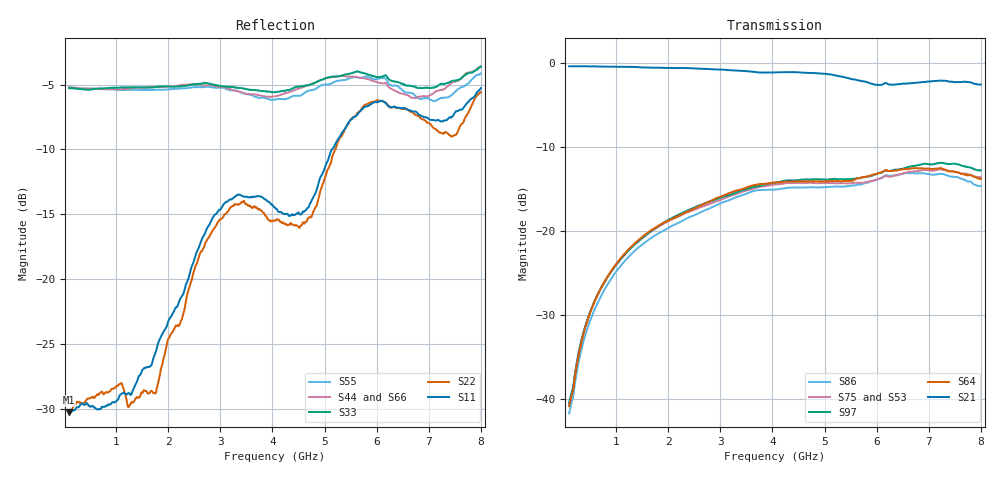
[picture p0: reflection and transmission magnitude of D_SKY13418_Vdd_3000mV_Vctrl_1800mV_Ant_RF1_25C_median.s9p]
# GHz S DB R 50
! THRU S21 mag phase subtraction.
! HALF_THRU
! EN33-165-011-v1_HALF_THRU_1 EN33-165-011-v1_HALF_THRU_2 EN33-165-011-v1_HALF_THRU_3 EN33-165-011-v1_HALF_THRU_4 EN33-165-011-v1_HALF_THRU_5 EN33-165-011-v1_HALF_THRU_6 EN33-165-011-v1_HALF_THRU_7 EN33-165-011-v1_HALF_THRU_8 EN33-165-011-v1_HALF_THRU_9
! THRU Ports: 1 2
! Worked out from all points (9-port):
!   801 points, 100 MHz to 8 GHz, reference 50 ohm
!   strongest paths, dB at 100 MHz, 2.075 GHz, 4.05 GHz, 6.025 GHz, 8 GHz:
!     S21: -0.4, -0.6, -1.1, -2.6, -2.5
!     S64: -40.8, -18.5, -14.2, -13.1, -13.8
!     S97: -40.5, -18.4, -14.2, -13.1, -12.8
!     S75: -40.6, -18.6, -14.4, -13.8, -13.5
!     S53: -41.0, -18.8, -14.6, -13.8, -13.6
!     S86: -41.7, -19.4, -15.0, -13.8, -14.6
!   lowest |S11| = -30.3 dB at 100 MHz (marker M1), VSWR 1.06, Z = 53.1 + j0.244 ohm
!   |S11| at or under -10 dB: start of sweep to 5.141 GHz
